| IBIS file stm32u535_545_lqfp100.ibs
[IBIS ver] 4.2
[File name] stm32u535_545_lqfp100.ibs
[File Rev] rev1.0
[Date]  11-09-2023
[Source] Data Created at STMicroelectronics
[Notes]  File originated from ELDO simulations.
[Disclaimer]  This information is for modeling purpose only and is
   not guaranteed. The information is subject to change without
   notice.
[Copyright] Copyright 2023 STMicroelectronics Inc.
|   Component stm32u535_545_lqfp100
[Component] stm32u535_545_lqfp100
[Manufacturer] STMicroelectronics
[Package]
| variable   typ   min   max
R_pkg  0  NA  NA
L_pkg  0  NA  NA
C_pkg  0  NA  NA
[Pin]   signal_name   model_name
1  PE2  io8_100m_hslv_ft
2  PE3  io8_100m_hslv_tamp_ft
3  PE4  io8_100m_hslv_tamp_ft
4  PE5  io8_100m_hslv_tamp_ft
5  PE6  io8_100m_hslv_tamp_ft
6  VBAT  power
7  PC13  io8_100m_ft_v33
8  PC14-OSC32_IN  io8_100m_tamp_ft
9  PC15-OSC32_OUT  io8_100m_tamp_ft
10  VSS  gnd
11  VDD  power
12  PH0-OSC_IN  io8_100m_ft
13  PH1-OSC_OUT  io8_100m_ft
14  NRST  nc
15  PC0  io8_100m_hslv_i2c_ft
16  PC1  io8_166m_hslv_i2c_ft
17  PC2  io8_100m_hslv_ft
18  PC3  io8_100m_hslv_ft
19  VSSA  nc
20  VREFM  nc
21  VREFP  nc
22  VDDA  power
23  PA0  io8_100m_hslv_tamp_ft
24  PA1  io8_100m_hslv_tamp_ft
25  PA2  io8_100m_hslv_ft
26  PA3  io8_166m_hslv_ft
27  VSS  gnd
28  VDD  power
29  PA4  io8_100m_hslv_ft
30  PA5  io8_100m_ft
31  PA6  io8_100m_hslv_ft
32  PA7  io8_100m_hslv_i2c_ft
33  PC4  io8_100m_hslv_ft
34  PC5  io8_100m_tamp_ft
35  PB0  io8_100m_hslv_ft
36  PB1  io8_100m_hslv_ft
37  PB2  io8_100m_hslv_tamp_ft
38  PE7  io8_100m_hslv_ft
39  PE8  io8_100m_hslv_ft
40  PE9  io8_166m_hslv_ft
41  PE10  io8_166m_hslv_ft
42  PE11  io8_100m_hslv_ft
43  PE12  io8_100m_hslv_ft
44  PE13  io8_100m_hslv_ft
45  PE14  io8_100m_hslv_ft
46  PE15  io8_100m_hslv_ft
47  PB10  io8_166m_hslv_i2c_ft
48  VCAP  nc
49  VSS  gnd
50  VDD  power
51  PB12  io8_166m_hslv_ft
52  PB13  io8_100m_i2c_ft
53  PB14  io8_100m_i2c_ft
54  PB15  io8_100m_ft
55  PD8  io8_100m_hslv_ft
56  PD9  io8_100m_hslv_ft
57  PD10  io8_100m_hslv_ft
58  PD11  io8_100m_hslv_ft
59  PD12  io8_100m_hslv_i2c_ft
60  PD13  io8_100m_hslv_i2c_ft
61  PD14  io8_100m_hslv_ft
62  PD15  io8_100m_hslv_ft
63  PC6  io8_100m_hslv_ft
64  PC7  io8_100m_hslv_ft
65  PC8  io8_100m_hslv_ft
66  PC9  io8_100m_hslv_ft
67  PA8  io8_166m_hslv_ft
68  PA9  io8_100m_ft
69  PA10  io8_100m_ft
70  PA11  io8_usb_ft
71  PA12  io8_usb_ft
72  PA13  io8_100m_ft
73  VDDUSB  power
74  VSS  gnd
75  VDD  power
76  PA14  io8_100m_ft
77  PA15  io8_100m_ft
78  PC10  io8_100m_hslv_ft
79  PC11  io8_100m_hslv_ft
80  PC12  io8_166m_hslv_ft
81  PD0  io8_100m_hslv_ft
82  PD1  io8_100m_hslv_ft
83  PD2  io8_100m_hslv_ft
84  PD3  io8_166m_hslv_ft
85  PD4  io8_100m_hslv_ft
86  PD5  io8_100m_hslv_ft
87  PD6  io8_166m_hslv_ft
88  PD7  io8_100m_hslv_ft
89  PB3  io8_100m_i2c_ft
90  PB4  io8_100m_i2c_ft
91  PB5  io8_166m_hslv_ft
92  PB6  io8_100m_i2c_ft
93  PB7  io8_166m_hslv_i2c_ft
94  PH3-BOOT0  io8_100m_ft
95  PB8  io8_100m_hslv_i2c_ft
96  PB9  io8_100m_hslv_i2c_ft
97  PE0  io8_100m_hslv_ft
98  PE1  io8_100m_hslv_ft
99  VSS  gnd
100  VDD power
[Package Model]   455-lqfp-14x14-100-ldo-230504
[Pin Mapping]   pulldown_ref   pullup_ref   | Comment
1  gndio  vddiom
2  gndio  vddiom
3  gndio  vddiom
4  gndio  vddiom
5  gndio  vddiom
6  nc  vsw
7  gndio  vddiom  | Depending on IO usage
| 7  gndio  vsw  | Depending on IO usage
8  gndio  vddiom  | Depending on IO usage
| 8  gndio  vsw  | Depending on IO usage
9  gndio  vddiom  | Depending on IO usage
| 9  gndio  vsw  | Depending on IO usage
10  gndio  nc
11  nc  vddiom
12  gndio  vddiom
13  gndio  vddiom
14  nc   nc
15  gndio  vddiom
16  gndio  vddiom
17  gndio  vddiom
18  gndio  vddiom
19  nc  nc
20  nc  nc
21  nc  nc
22  nc  vddiom
23  gndio  vddiom
24  gndio  vddiom
25  gndio  vddiom
26  gndio  vddiom
27  gndio  nc
28  nc  vddiom
29  gndio  vddiom
30  gndio  vddiom
31  gndio  vddiom
32  gndio  vddiom
33  gndio  vddiom
34  gndio  vddiom
35  gndio  vddiom
36  gndio  vddiom
37  gndio  vddiom
38  gndio  vddiom
39  gndio  vddiom
40  gndio  vddiom
41  gndio  vddiom
42  gndio  vddiom
43  gndio  vddiom
44  gndio  vddiom
45  gndio  vddiom
46  gndio  vddiom
47  gndio  vddiom
48  nc  nc
49  gndio  nc
50  nc  vddiom
51  gndio  vddiom
52  gndio  vddiom
53  gndio  vddiom
54  gndio  vddiom
55  gndio  vddiom
56  gndio  vddiom
57  gndio  vddiom
58  gndio  vddiom
59  gndio  vddiom
60  gndio  vddiom
61  gndio  vddiom
62  gndio  vddiom
63  gndio  vddiom
64  gndio  vddiom
65  gndio  vddiom
66  gndio  vddiom
67  gndio  vddiom
68  gndio  vddiom  | Depending on IO usage
| 68  gndio  vddusb  | Depending on IO usage
69  gndio  vddiom  | Depending on IO usage
| 69  gndio  vddusb  | Depending on IO usage
70  gndio  vddiom  | Depending on IO usage
| 70  gndio  vddusb  | Depending on IO usage
71  gndio  vddiom  | Depending on IO usage
| 71  gndio  vddusb  | Depending on IO usage
72  gndio  vddiom  | Depending on IO usage
| 72  gndio  vddusb  | Depending on IO usage
73  nc  vddusb
74  gndio  nc
75  nc  vddiom
76  gndio  vddiom
77  gndio  vddiom
78  gndio  vddiom
79  gndio  vddiom
80  gndio  vddiom
81  gndio  vddiom
82  gndio  vddiom
83  gndio  vddiom
84  gndio  vddiom
85  gndio  vddiom
86  gndio  vddiom
87  gndio  vddiom
88  gndio  vddiom
89  gndio  vddiom
90  gndio  vddiom
91  gndio  vddiom
92  gndio  vddiom
93  gndio  vddiom
94  gndio  vddiom
95  gndio  vddiom
96  gndio  vddiom
97  gndio  vddiom
98  gndio  vddiom
99  gndio  nc
100  nc  vddiom
[Model Selector] io8_100m_ft
io8_100m_ft_hs_1v2  "IO8_FT 100MHz high speed @ 1.2V"
io8_100m_ft_fs_1v2  "IO8_FT 100MHz fast speed @ 1.2V"
io8_100m_ft_fs_pd_1v2  "IO8_FT 100MHz fast speed @ 1.2V pulldown"
io8_100m_ft_ms_1v2  "IO8_FT 100MHz med speed @ 1.2V"
io8_100m_ft_ms_pd_1v2  "IO8_FT 100MHz med speed @ 1.2V pulldown"
io8_100m_ft_ls_1v2  "IO8_FT 100MHz low speed @ 1.2V"
io8_100m_ft_ls_pd_1v2  "IO8_FT 100MHz low speed @ 1.2V pulldown"
io8_100m_ft_hs_1v8  "IO8_FT 100MHz high speed @ 1.8V"
io8_100m_ft_hs_pd_1v8  "IO8_FT 100MHz high speed @ 1.8V pulldown"
io8_100m_ft_fs_1v8  "IO8_FT 100MHz fast speed @ 1.8V"
io8_100m_ft_fs_pd_1v8  "IO8_FT 100MHz fast speed @ 1.8V pulldown"
io8_100m_ft_ms_1v8  "IO8_FT 100MHz med speed @ 1.8V"
io8_100m_ft_ms_pd_1v8  "IO8_FT 100MHz med speed @ 1.8V pulldown"
io8_100m_ft_ls_1v8  "IO8_FT 100MHz low speed @ 1.8V"
io8_100m_ft_ls_pd_1v8  "IO8_FT 100MHz low speed @ 1.8V pulldown"
io8_100m_ft_hs_3v3  "IO8_FT 100MHz high speed @ 3.3V"
io8_100m_ft_hs_pd_3v3  "IO8_FT 100MHz high speed @ 3.3V pulldown"
io8_100m_ft_fs_3v3  "IO8_FT 100MHz fast speed @ 3.3V"
io8_100m_ft_fs_pd_3v3  "IO8_FT 100MHz fast speed @ 3.3V pulldown"
io8_100m_ft_ms_3v3  "IO8_FT 100MHz med speed @ 3.3V"
io8_100m_ft_ms_pd_3v3  "IO8_FT 100MHz med speed @ 3.3V pulldown"
io8_100m_ft_ls_3v3  "IO8_FT 100MHz low speed @ 3.3V"
io8_100m_ft_ls_pd_3v3  "IO8_FT 100MHz low speed @ 3.3V pulldown"
[Model Selector] io8_100m_hslv_ft
io8_100m_ft_hs_1v2  "IO8_FT 100MHz high speed @ 1.2V"
io8_100m_ft_hs_pu_1v2  "IO8_FT 100MHz high speed @ 1.2V pullup"
io8_100m_ft_hs_pd_1v2  "IO8_FT 100MHz high speed @ 1.2V pulldown"
io8_100m_ft_fs_1v2  "IO8_FT 100MHz fast speed @ 1.2V"
io8_100m_ft_fs_pu_1v2  "IO8_FT 100MHz fast speed @ 1.2V pullup"
io8_100m_ft_fs_pd_1v2  "IO8_FT 100MHz fast speed @ 1.2V pulldown"
io8_100m_ft_ms_1v2  "IO8_FT 100MHz med speed @ 1.2V"
io8_100m_ft_ms_pu_1v2  "IO8_FT 100MHz med speed @ 1.2V pullup"
io8_100m_ft_ms_pd_1v2  "IO8_FT 100MHz med speed @ 1.2V pulldown"
io8_100m_ft_ls_1v2  "IO8_FT 100MHz low speed @ 1.2V"
io8_100m_ft_ls_pu_1v2  "IO8_FT 100MHz low speed @ 1.2V pullup"
io8_100m_ft_ls_pd_1v2  "IO8_FT 100MHz low speed @ 1.2V pulldown"
io8_100m_ft_hs_1v8  "IO8_FT 100MHz high speed @ 1.8V"
io8_100m_ft_hs_pu_1v8  "IO8_FT 100MHz high speed @ 1.8V pullup"
io8_100m_ft_hs_pd_1v8  "IO8_FT 100MHz high speed @ 1.8V pulldown"
io8_100m_ft_fs_1v8  "IO8_FT 100MHz fast speed @ 1.8V"
io8_100m_ft_fs_pu_1v8  "IO8_FT 100MHz fast speed @ 1.8V pullup"
io8_100m_ft_fs_pd_1v8  "IO8_FT 100MHz fast speed @ 1.8V pulldown"
io8_100m_ft_ms_1v8  "IO8_FT 100MHz med speed @ 1.8V"
io8_100m_ft_ms_pu_1v8  "IO8_FT 100MHz med speed @ 1.8V pullup"
io8_100m_ft_ms_pd_1v8  "IO8_FT 100MHz med speed @ 1.8V pulldown"
io8_100m_ft_ls_1v8  "IO8_FT 100MHz low speed @ 1.8V"
io8_100m_ft_ls_pu_1v8  "IO8_FT 100MHz low speed @ 1.8V pullup"
io8_100m_ft_ls_pd_1v8  "IO8_FT 100MHz low speed @ 1.8V pulldown"
io8_100m_ft_hs_3v3  "IO8_FT 100MHz high speed @ 3.3V"
io8_100m_ft_hs_pu_3v3  "IO8_FT 100MHz high speed @ 3.3V pullup"
io8_100m_ft_hs_pd_3v3  "IO8_FT 100MHz high speed @ 3.3V pulldown"
io8_100m_ft_fs_3v3  "IO8_FT 100MHz fast speed @ 3.3V"
io8_100m_ft_fs_pu_3v3  "IO8_FT 100MHz fast speed @ 3.3V pullup"
io8_100m_ft_fs_pd_3v3  "IO8_FT 100MHz fast speed @ 3.3V pulldown"
io8_100m_ft_ms_3v3  "IO8_FT 100MHz med speed @ 3.3V"
io8_100m_ft_ms_pu_3v3  "IO8_FT 100MHz med speed @ 3.3V pullup"
io8_100m_ft_ms_pd_3v3  "IO8_FT 100MHz med speed @ 3.3V pulldown"
io8_100m_ft_ls_3v3  "IO8_FT 100MHz low speed @ 3.3V"
io8_100m_ft_ls_pu_3v3  "IO8_FT 100MHz low speed @ 3.3V pullup"
io8_100m_ft_ls_pd_3v3  "IO8_FT 100MHz low speed @ 3.3V pulldown"
io8_100m_hslv_ft_hs_1v2  "IO8_FT 100MHz HSLV high speed @ 1.2V"
io8_100m_hslv_ft_hs_pu_1v2  "IO8_FT 100MHz HSLV high speed @ 1.2V pullup"
io8_100m_hslv_ft_hs_pd_1v2  "IO8_FT 100MHz HSLV high speed @ 1.2V pulldown"
io8_100m_hslv_ft_fs_1v2  "IO8_FT 100MHz HSLV fast speed @ 1.2V"
io8_100m_hslv_ft_fs_pu_1v2  "IO8_FT 100MHz HSLV fast speed @ 1.2V pullup"
io8_100m_hslv_ft_fs_pd_1v2  "IO8_FT 100MHz HSLV fast speed @ 1.2V pulldown"
io8_100m_hslv_ft_ms_1v2  "IO8_FT 100MHz HSLV med speed @ 1.2V"
io8_100m_hslv_ft_ms_pu_1v2  "IO8_FT 100MHz HSLV med speed @ 1.2V pullup"
io8_100m_hslv_ft_ms_pd_1v2  "IO8_FT 100MHz HSLV med speed @ 1.2V pulldown"
io8_100m_hslv_ft_ls_1v2  "IO8_FT 100MHz HSLV low speed @ 1.2V"
io8_100m_hslv_ft_ls_pu_1v2  "IO8_FT 100MHz HSLV low speed @ 1.2V pullup"
io8_100m_hslv_ft_ls_pd_1v2  "IO8_FT 100MHz HSLV low speed @ 1.2V pulldown"
io8_100m_hslv_ft_hs_1v8  "IO8_FT 100MHz HSLV high speed @ 1.8V"
io8_100m_hslv_ft_hs_pu_1v8  "IO8_FT 100MHz HSLV high speed @ 1.8V pullup"
io8_100m_hslv_ft_hs_pd_1v8  "IO8_FT 100MHz HSLV high speed @ 1.8V pulldown"
io8_100m_hslv_ft_fs_1v8  "IO8_FT 100MHz HSLV fast speed @ 1.8V"
io8_100m_hslv_ft_fs_pu_1v8  "IO8_FT 100MHz HSLV fast speed @ 1.8V pullup"
io8_100m_hslv_ft_fs_pd_1v8  "IO8_FT 100MHz HSLV fast speed @ 1.8V pulldown"
io8_100m_hslv_ft_ms_1v8  "IO8_FT 100MHz HSLV med speed @ 1.8V"
io8_100m_hslv_ft_ms_pu_1v8  "IO8_FT 100MHz HSLV med speed @ 1.8V pullup"
io8_100m_hslv_ft_ms_pd_1v8  "IO8_FT 100MHz HSLV med speed @ 1.8V pulldown"
io8_100m_hslv_ft_ls_1v8  "IO8_FT 100MHz HSLV low speed @ 1.8V"
io8_100m_hslv_ft_ls_pu_1v8  "IO8_FT 100MHz HSLV low speed @ 1.8V pullup"
io8_100m_hslv_ft_ls_pd_1v8  "IO8_FT 100MHz HSLV low speed @ 1.8V pulldown"
io8_100m_hslv_ft_hs_2v5  "IO8_FT 100MHz HSLV high speed @ 2.5V"
io8_100m_hslv_ft_hs_pu_2v5  "IO8_FT 100MHz HSLV high speed @ 2.5V pullup"
io8_100m_hslv_ft_hs_pd_2v5  "IO8_FT 100MHz HSLV high speed @ 2.5V pulldown"
io8_100m_hslv_ft_fs_2v5  "IO8_FT 100MHz HSLV fast speed @ 2.5V"
io8_100m_hslv_ft_fs_pu_2v5  "IO8_FT 100MHz HSLV fast speed @ 2.5V pullup"
io8_100m_hslv_ft_fs_pd_2v5  "IO8_FT 100MHz HSLV fast speed @ 2.5V pulldown"
io8_100m_hslv_ft_ms_2v5  "IO8_FT 100MHz HSLV med speed @ 2.5V"
io8_100m_hslv_ft_ms_pu_2v5  "IO8_FT 100MHz HSLV med speed @ 2.5V pullup"
io8_100m_hslv_ft_ms_pd_2v5  "IO8_FT 100MHz HSLV med speed @ 2.5V pulldown"
io8_100m_hslv_ft_ls_2v5  "IO8_FT 100MHz HSLV low speed @ 2.5V"
io8_100m_hslv_ft_ls_pu_2v5  "IO8_FT 100MHz HSLV low speed @ 2.5V pullup"
io8_100m_hslv_ft_ls_pd_2v5  "IO8_FT 100MHz HSLV low speed @ 2.5V pulldown"
[Model Selector] io8_100m_hslv_i2c_ft
io8_100m_ft_hs_1v2  "IO8_FT 100MHz high speed @ 1.2V"
io8_100m_ft_hs_pu_1v2  "IO8_FT 100MHz high speed @ 1.2V pullup"
io8_100m_ft_hs_pd_1v2  "IO8_FT 100MHz high speed @ 1.2V pulldown"
io8_100m_ft_fs_1v2  "IO8_FT 100MHz fast speed @ 1.2V"
io8_100m_ft_fs_pu_1v2  "IO8_FT 100MHz fast speed @ 1.2V pullup"
io8_100m_ft_fs_pd_1v2  "IO8_FT 100MHz fast speed @ 1.2V pulldown"
io8_100m_ft_ms_1v2  "IO8_FT 100MHz med speed @ 1.2V"
io8_100m_ft_ms_pu_1v2  "IO8_FT 100MHz med speed @ 1.2V pullup"
io8_100m_ft_ms_pd_1v2  "IO8_FT 100MHz med speed @ 1.2V pulldown"
io8_100m_ft_ls_1v2  "IO8_FT 100MHz low speed @ 1.2V"
io8_100m_ft_ls_pu_1v2  "IO8_FT 100MHz low speed @ 1.2V pullup"
io8_100m_ft_ls_pd_1v2  "IO8_FT 100MHz low speed @ 1.2V pulldown"
io8_100m_ft_hs_1v8  "IO8_FT 100MHz high speed @ 1.8V"
io8_100m_ft_hs_pu_1v8  "IO8_FT 100MHz high speed @ 1.8V pullup"
io8_100m_ft_hs_pd_1v8  "IO8_FT 100MHz high speed @ 1.8V pulldown"
io8_100m_ft_fs_1v8  "IO8_FT 100MHz fast speed @ 1.8V"
io8_100m_ft_fs_pu_1v8  "IO8_FT 100MHz fast speed @ 1.8V pullup"
io8_100m_ft_fs_pd_1v8  "IO8_FT 100MHz fast speed @ 1.8V pulldown"
io8_100m_ft_ms_1v8  "IO8_FT 100MHz med speed @ 1.8V"
io8_100m_ft_ms_pu_1v8  "IO8_FT 100MHz med speed @ 1.8V pullup"
io8_100m_ft_ms_pd_1v8  "IO8_FT 100MHz med speed @ 1.8V pulldown"
io8_100m_ft_ls_1v8  "IO8_FT 100MHz low speed @ 1.8V"
io8_100m_ft_ls_pu_1v8  "IO8_FT 100MHz low speed @ 1.8V pullup"
io8_100m_ft_ls_pd_1v8  "IO8_FT 100MHz low speed @ 1.8V pulldown"
io8_100m_ft_hs_3v3  "IO8_FT 100MHz high speed @ 3.3V"
io8_100m_ft_hs_pu_3v3  "IO8_FT 100MHz high speed @ 3.3V pullup"
io8_100m_ft_hs_pd_3v3  "IO8_FT 100MHz high speed @ 3.3V pulldown"
io8_100m_ft_fs_3v3  "IO8_FT 100MHz fast speed @ 3.3V"
io8_100m_ft_fs_pu_3v3  "IO8_FT 100MHz fast speed @ 3.3V pullup"
io8_100m_ft_fs_pd_3v3  "IO8_FT 100MHz fast speed @ 3.3V pulldown"
io8_100m_ft_ms_3v3  "IO8_FT 100MHz med speed @ 3.3V"
io8_100m_ft_ms_pu_3v3  "IO8_FT 100MHz med speed @ 3.3V pullup"
io8_100m_ft_ms_pd_3v3  "IO8_FT 100MHz med speed @ 3.3V pulldown"
io8_100m_ft_ls_3v3  "IO8_FT 100MHz low speed @ 3.3V"
io8_100m_ft_ls_pu_3v3  "IO8_FT 100MHz low speed @ 3.3V pullup"
io8_100m_ft_ls_pd_3v3  "IO8_FT 100MHz low speed @ 3.3V pulldown"
io8_100m_hslv_ft_hs_1v2  "IO8_FT 100MHz HSLV high speed @ 1.2V"
io8_100m_hslv_ft_hs_pu_1v2  "IO8_FT 100MHz HSLV high speed @ 1.2V pullup"
io8_100m_hslv_ft_hs_pd_1v2  "IO8_FT 100MHz HSLV high speed @ 1.2V pulldown"
io8_100m_hslv_ft_fs_1v2  "IO8_FT 100MHz HSLV fast speed @ 1.2V"
io8_100m_hslv_ft_fs_pu_1v2  "IO8_FT 100MHz HSLV fast speed @ 1.2V pullup"
io8_100m_hslv_ft_fs_pd_1v2  "IO8_FT 100MHz HSLV fast speed @ 1.2V pulldown"
io8_100m_hslv_ft_ms_1v2  "IO8_FT 100MHz HSLV med speed @ 1.2V"
io8_100m_hslv_ft_ms_pu_1v2  "IO8_FT 100MHz HSLV med speed @ 1.2V pullup"
io8_100m_hslv_ft_ms_pd_1v2  "IO8_FT 100MHz HSLV med speed @ 1.2V pulldown"
io8_100m_hslv_ft_ls_1v2  "IO8_FT 100MHz HSLV low speed @ 1.2V"
io8_100m_hslv_ft_ls_pu_1v2  "IO8_FT 100MHz HSLV low speed @ 1.2V pullup"
io8_100m_hslv_ft_ls_pd_1v2  "IO8_FT 100MHz HSLV low speed @ 1.2V pulldown"
io8_100m_hslv_ft_hs_1v8  "IO8_FT 100MHz HSLV high speed @ 1.8V"
io8_100m_hslv_ft_hs_pu_1v8  "IO8_FT 100MHz HSLV high speed @ 1.8V pullup"
io8_100m_hslv_ft_hs_pd_1v8  "IO8_FT 100MHz HSLV high speed @ 1.8V pulldown"
io8_100m_hslv_ft_fs_1v8  "IO8_FT 100MHz HSLV fast speed @ 1.8V"
io8_100m_hslv_ft_fs_pu_1v8  "IO8_FT 100MHz HSLV fast speed @ 1.8V pullup"
io8_100m_hslv_ft_fs_pd_1v8  "IO8_FT 100MHz HSLV fast speed @ 1.8V pulldown"
io8_100m_hslv_ft_ms_1v8  "IO8_FT 100MHz HSLV med speed @ 1.8V"
io8_100m_hslv_ft_ms_pu_1v8  "IO8_FT 100MHz HSLV med speed @ 1.8V pullup"
io8_100m_hslv_ft_ms_pd_1v8  "IO8_FT 100MHz HSLV med speed @ 1.8V pulldown"
io8_100m_hslv_ft_ls_1v8  "IO8_FT 100MHz HSLV low speed @ 1.8V"
io8_100m_hslv_ft_ls_pu_1v8  "IO8_FT 100MHz HSLV low speed @ 1.8V pullup"
io8_100m_hslv_ft_ls_pd_1v8  "IO8_FT 100MHz HSLV low speed @ 1.8V pulldown"
io8_100m_hslv_ft_hs_2v5  "IO8_FT 100MHz HSLV high speed @ 2.5V"
io8_100m_hslv_ft_hs_pu_2v5  "IO8_FT 100MHz HSLV high speed @ 2.5V pullup"
io8_100m_hslv_ft_hs_pd_2v5  "IO8_FT 100MHz HSLV high speed @ 2.5V pulldown"
io8_100m_hslv_ft_fs_2v5  "IO8_FT 100MHz HSLV fast speed @ 2.5V"
io8_100m_hslv_ft_fs_pu_2v5  "IO8_FT 100MHz HSLV fast speed @ 2.5V pullup"
io8_100m_hslv_ft_fs_pd_2v5  "IO8_FT 100MHz HSLV fast speed @ 2.5V pulldown"
io8_100m_hslv_ft_ms_2v5  "IO8_FT 100MHz HSLV med speed @ 2.5V"
io8_100m_hslv_ft_ms_pu_2v5  "IO8_FT 100MHz HSLV med speed @ 2.5V pullup"
io8_100m_hslv_ft_ms_pd_2v5  "IO8_FT 100MHz HSLV med speed @ 2.5V pulldown"
io8_100m_hslv_ft_ls_2v5  "IO8_FT 100MHz HSLV low speed @ 2.5V"
io8_100m_hslv_ft_ls_pu_2v5  "IO8_FT 100MHz HSLV low speed @ 2.5V pullup"
io8_100m_hslv_ft_ls_pd_2v5  "IO8_FT 100MHz HSLV low speed @ 2.5V pulldown"
[Model Selector] io8_100m_hslv_tamp_ft
io8_100m_ft_hs_1v2  "IO8_FT 100MHz high speed @ 1.2V"
io8_100m_ft_hs_pu_1v2  "IO8_FT 100MHz high speed @ 1.2V pullup"
io8_100m_ft_hs_pd_1v2  "IO8_FT 100MHz high speed @ 1.2V pulldown"
io8_100m_ft_fs_1v2  "IO8_FT 100MHz fast speed @ 1.2V"
io8_100m_ft_fs_pu_1v2  "IO8_FT 100MHz fast speed @ 1.2V pullup"
io8_100m_ft_fs_pd_1v2  "IO8_FT 100MHz fast speed @ 1.2V pulldown"
io8_100m_ft_ms_1v2  "IO8_FT 100MHz med speed @ 1.2V"
io8_100m_ft_ms_pu_1v2  "IO8_FT 100MHz med speed @ 1.2V pullup"
io8_100m_ft_ms_pd_1v2  "IO8_FT 100MHz med speed @ 1.2V pulldown"
io8_100m_ft_ls_1v2  "IO8_FT 100MHz low speed @ 1.2V"
io8_100m_ft_ls_pu_1v2  "IO8_FT 100MHz low speed @ 1.2V pullup"
io8_100m_ft_ls_pd_1v2  "IO8_FT 100MHz low speed @ 1.2V pulldown"
io8_100m_ft_hs_1v8  "IO8_FT 100MHz high speed @ 1.8V"
io8_100m_ft_hs_pu_1v8  "IO8_FT 100MHz high speed @ 1.8V pullup"
io8_100m_ft_hs_pd_1v8  "IO8_FT 100MHz high speed @ 1.8V pulldown"
io8_100m_ft_fs_1v8  "IO8_FT 100MHz fast speed @ 1.8V"
io8_100m_ft_fs_pu_1v8  "IO8_FT 100MHz fast speed @ 1.8V pullup"
io8_100m_ft_fs_pd_1v8  "IO8_FT 100MHz fast speed @ 1.8V pulldown"
io8_100m_ft_ms_1v8  "IO8_FT 100MHz med speed @ 1.8V"
io8_100m_ft_ms_pu_1v8  "IO8_FT 100MHz med speed @ 1.8V pullup"
io8_100m_ft_ms_pd_1v8  "IO8_FT 100MHz med speed @ 1.8V pulldown"
io8_100m_ft_ls_1v8  "IO8_FT 100MHz low speed @ 1.8V"
io8_100m_ft_ls_pu_1v8  "IO8_FT 100MHz low speed @ 1.8V pullup"
io8_100m_ft_ls_pd_1v8  "IO8_FT 100MHz low speed @ 1.8V pulldown"
io8_100m_ft_hs_3v3  "IO8_FT 100MHz high speed @ 3.3V"
io8_100m_ft_hs_pu_3v3  "IO8_FT 100MHz high speed @ 3.3V pullup"
io8_100m_ft_hs_pd_3v3  "IO8_FT 100MHz high speed @ 3.3V pulldown"
io8_100m_ft_fs_3v3  "IO8_FT 100MHz fast speed @ 3.3V"
io8_100m_ft_fs_pu_3v3  "IO8_FT 100MHz fast speed @ 3.3V pullup"
io8_100m_ft_fs_pd_3v3  "IO8_FT 100MHz fast speed @ 3.3V pulldown"
io8_100m_ft_ms_3v3  "IO8_FT 100MHz med speed @ 3.3V"
io8_100m_ft_ms_pu_3v3  "IO8_FT 100MHz med speed @ 3.3V pullup"
io8_100m_ft_ms_pd_3v3  "IO8_FT 100MHz med speed @ 3.3V pulldown"
io8_100m_ft_ls_3v3  "IO8_FT 100MHz low speed @ 3.3V"
io8_100m_ft_ls_pu_3v3  "IO8_FT 100MHz low speed @ 3.3V pullup"
io8_100m_ft_ls_pd_3v3  "IO8_FT 100MHz low speed @ 3.3V pulldown"
io8_100m_hslv_ft_hs_1v2  "IO8_FT 100MHz HSLV high speed @ 1.2V"
io8_100m_hslv_ft_hs_pu_1v2  "IO8_FT 100MHz HSLV high speed @ 1.2V pullup"
io8_100m_hslv_ft_hs_pd_1v2  "IO8_FT 100MHz HSLV high speed @ 1.2V pulldown"
io8_100m_hslv_ft_fs_1v2  "IO8_FT 100MHz HSLV fast speed @ 1.2V"
io8_100m_hslv_ft_fs_pu_1v2  "IO8_FT 100MHz HSLV fast speed @ 1.2V pullup"
io8_100m_hslv_ft_fs_pd_1v2  "IO8_FT 100MHz HSLV fast speed @ 1.2V pulldown"
io8_100m_hslv_ft_ms_1v2  "IO8_FT 100MHz HSLV med speed @ 1.2V"
io8_100m_hslv_ft_ms_pu_1v2  "IO8_FT 100MHz HSLV med speed @ 1.2V pullup"
io8_100m_hslv_ft_ms_pd_1v2  "IO8_FT 100MHz HSLV med speed @ 1.2V pulldown"
io8_100m_hslv_ft_ls_1v2  "IO8_FT 100MHz HSLV low speed @ 1.2V"
io8_100m_hslv_ft_ls_pu_1v2  "IO8_FT 100MHz HSLV low speed @ 1.2V pullup"
io8_100m_hslv_ft_ls_pd_1v2  "IO8_FT 100MHz HSLV low speed @ 1.2V pulldown"
io8_100m_hslv_ft_hs_1v8  "IO8_FT 100MHz HSLV high speed @ 1.8V"
io8_100m_hslv_ft_hs_pu_1v8  "IO8_FT 100MHz HSLV high speed @ 1.8V pullup"
io8_100m_hslv_ft_hs_pd_1v8  "IO8_FT 100MHz HSLV high speed @ 1.8V pulldown"
io8_100m_hslv_ft_fs_1v8  "IO8_FT 100MHz HSLV fast speed @ 1.8V"
io8_100m_hslv_ft_fs_pu_1v8  "IO8_FT 100MHz HSLV fast speed @ 1.8V pullup"
io8_100m_hslv_ft_fs_pd_1v8  "IO8_FT 100MHz HSLV fast speed @ 1.8V pulldown"
io8_100m_hslv_ft_ms_1v8  "IO8_FT 100MHz HSLV med speed @ 1.8V"
io8_100m_hslv_ft_ms_pu_1v8  "IO8_FT 100MHz HSLV med speed @ 1.8V pullup"
io8_100m_hslv_ft_ms_pd_1v8  "IO8_FT 100MHz HSLV med speed @ 1.8V pulldown"
io8_100m_hslv_ft_ls_1v8  "IO8_FT 100MHz HSLV low speed @ 1.8V"
io8_100m_hslv_ft_ls_pu_1v8  "IO8_FT 100MHz HSLV low speed @ 1.8V pullup"
io8_100m_hslv_ft_ls_pd_1v8  "IO8_FT 100MHz HSLV low speed @ 1.8V pulldown"
io8_100m_hslv_ft_hs_2v5  "IO8_FT 100MHz HSLV high speed @ 2.5V"
io8_100m_hslv_ft_hs_pu_2v5  "IO8_FT 100MHz HSLV high speed @ 2.5V pullup"
io8_100m_hslv_ft_hs_pd_2v5  "IO8_FT 100MHz HSLV high speed @ 2.5V pulldown"
io8_100m_hslv_ft_fs_2v5  "IO8_FT 100MHz HSLV fast speed @ 2.5V"
io8_100m_hslv_ft_fs_pu_2v5  "IO8_FT 100MHz HSLV fast speed @ 2.5V pullup"
io8_100m_hslv_ft_fs_pd_2v5  "IO8_FT 100MHz HSLV fast speed @ 2.5V pulldown"
io8_100m_hslv_ft_ms_2v5  "IO8_FT 100MHz HSLV med speed @ 2.5V"
io8_100m_hslv_ft_ms_pu_2v5  "IO8_FT 100MHz HSLV med speed @ 2.5V pullup"
io8_100m_hslv_ft_ms_pd_2v5  "IO8_FT 100MHz HSLV med speed @ 2.5V pulldown"
io8_100m_hslv_ft_ls_2v5  "IO8_FT 100MHz HSLV low speed @ 2.5V"
io8_100m_hslv_ft_ls_pu_2v5  "IO8_FT 100MHz HSLV low speed @ 2.5V pullup"
io8_100m_hslv_ft_ls_pd_2v5  "IO8_FT 100MHz HSLV low speed @ 2.5V pulldown"
io8_ft_v33_hs_1v2  "IO8_FT_V33 high speed @ 1.2V"
io8_ft_v33_hs_pu_1v2  "IO8_FT_V33 high speed @ 1.2V pullup"
io8_ft_v33_hs_pd_1v2  "IO8_FT_V33 high speed @ 1.2V pulldown"
io8_ft_v33_fs_1v2  "IO8_FT_V33 fast speed @ 1.2V"
io8_ft_v33_fs_pu_1v2  "IO8_FT_V33 fast speed @ 1.2V pullup"
io8_ft_v33_fs_pd_1v2  "IO8_FT_V33 fast speed @ 1.2V pulldown"
io8_ft_v33_ms_1v2  "IO8_FT_V33 med speed @ 1.2V"
io8_ft_v33_ms_pu_1v2  "IO8_FT_V33 med speed @ 1.2V pullup"
io8_ft_v33_ms_pd_1v2  "IO8_FT_V33 med speed @ 1.2V pulldown"
io8_ft_v33_ls_1v2  "IO8_FT_V33 low speed @ 1.2V"
io8_ft_v33_ls_pu_1v2  "IO8_FT_V33 low speed @ 1.2V pullup"
io8_ft_v33_ls_pd_1v2  "IO8_FT_V33 low speed @ 1.2V pulldown"
io8_ft_v33_hs_1v8  "IO8_FT_V33 high speed @ 1.8V"
io8_ft_v33_hs_pu_1v8  "IO8_FT_V33 high speed @ 1.8V pullup"
io8_ft_v33_hs_pd_1v8  "IO8_FT_V33 high speed @ 1.8V pulldown"
io8_ft_v33_fs_1v8  "IO8_FT_V33 fast speed @ 1.8V"
io8_ft_v33_fs_pu_1v8  "IO8_FT_V33 fast speed @ 1.8V pullup"
io8_ft_v33_fs_pd_1v8  "IO8_FT_V33 fast speed @ 1.8V pulldown"
io8_ft_v33_ms_1v8  "IO8_FT_V33 med speed @ 1.8V"
io8_ft_v33_ms_pu_1v8  "IO8_FT_V33 med speed @ 1.8V pullup"
io8_ft_v33_ms_pd_1v8  "IO8_FT_V33 med speed @ 1.8V pulldown"
io8_ft_v33_ls_1v8  "IO8_FT_V33 low speed @ 1.8V"
io8_ft_v33_ls_pu_1v8  "IO8_FT_V33 low speed @ 1.8V pullup"
io8_ft_v33_ls_pd_1v8  "IO8_FT_V33 low speed @ 1.8V pulldown"
io8_ft_v33_hs_3v3  "IO8_FT_V33 high speed @ 3.3V"
io8_ft_v33_hs_pu_3v3  "IO8_FT_V33 high speed @ 3.3V pullup"
io8_ft_v33_hs_pd_3v3  "IO8_FT_V33 high speed @ 3.3V pulldown"
io8_ft_v33_fs_3v3  "IO8_FT_V33 fast speed @ 3.3V"
io8_ft_v33_fs_pu_3v3  "IO8_FT_V33 fast speed @ 3.3V pullup"
io8_ft_v33_fs_pd_3v3  "IO8_FT_V33 fast speed @ 3.3V pulldown"
io8_ft_v33_ms_3v3  "IO8_FT_V33 med speed @ 3.3V"
io8_ft_v33_ms_pu_3v3  "IO8_FT_V33 med speed @ 3.3V pullup"
io8_ft_v33_ms_pd_3v3  "IO8_FT_V33 med speed @ 3.3V pulldown"
io8_ft_v33_ls_3v3  "IO8_FT_V33 low speed @ 3.3V"
io8_ft_v33_ls_pu_3v3  "IO8_FT_V33 low speed @ 3.3V pullup"
io8_ft_v33_ls_pd_3v3  "IO8_FT_V33 low speed @ 3.3V pulldown"
[Model Selector] io8_100m_i2c_ft
io8_100m_ft_hs_1v2  "IO8_FT 100MHz high speed @ 1.2V"
io8_100m_ft_hs_pu_1v2  "IO8_FT 100MHz high speed @ 1.2V pullup"
io8_100m_ft_hs_pd_1v2  "IO8_FT 100MHz high speed @ 1.2V pulldown"
io8_100m_ft_fs_1v2  "IO8_FT 100MHz fast speed @ 1.2V"
io8_100m_ft_fs_pu_1v2  "IO8_FT 100MHz fast speed @ 1.2V pullup"
io8_100m_ft_fs_pd_1v2  "IO8_FT 100MHz fast speed @ 1.2V pulldown"
io8_100m_ft_ms_1v2  "IO8_FT 100MHz med speed @ 1.2V"
io8_100m_ft_ms_pu_1v2  "IO8_FT 100MHz med speed @ 1.2V pullup"
io8_100m_ft_ms_pd_1v2  "IO8_FT 100MHz med speed @ 1.2V pulldown"
io8_100m_ft_ls_1v2  "IO8_FT 100MHz low speed @ 1.2V"
io8_100m_ft_ls_pu_1v2  "IO8_FT 100MHz low speed @ 1.2V pullup"
io8_100m_ft_ls_pd_1v2  "IO8_FT 100MHz low speed @ 1.2V pulldown"
io8_100m_ft_hs_1v8  "IO8_FT 100MHz high speed @ 1.8V"
io8_100m_ft_hs_pu_1v8  "IO8_FT 100MHz high speed @ 1.8V pullup"
io8_100m_ft_hs_pd_1v8  "IO8_FT 100MHz high speed @ 1.8V pulldown"
io8_100m_ft_fs_1v8  "IO8_FT 100MHz fast speed @ 1.8V"
io8_100m_ft_fs_pu_1v8  "IO8_FT 100MHz fast speed @ 1.8V pullup"
io8_100m_ft_fs_pd_1v8  "IO8_FT 100MHz fast speed @ 1.8V pulldown"
io8_100m_ft_ms_1v8  "IO8_FT 100MHz med speed @ 1.8V"
io8_100m_ft_ms_pu_1v8  "IO8_FT 100MHz med speed @ 1.8V pullup"
io8_100m_ft_ms_pd_1v8  "IO8_FT 100MHz med speed @ 1.8V pulldown"
io8_100m_ft_ls_1v8  "IO8_FT 100MHz low speed @ 1.8V"
io8_100m_ft_ls_pu_1v8  "IO8_FT 100MHz low speed @ 1.8V pullup"
io8_100m_ft_ls_pd_1v8  "IO8_FT 100MHz low speed @ 1.8V pulldown"
io8_100m_ft_hs_3v3  "IO8_FT 100MHz high speed @ 3.3V"
io8_100m_ft_hs_pu_3v3  "IO8_FT 100MHz high speed @ 3.3V pullup"
io8_100m_ft_hs_pd_3v3  "IO8_FT 100MHz high speed @ 3.3V pulldown"
io8_100m_ft_fs_3v3  "IO8_FT 100MHz fast speed @ 3.3V"
io8_100m_ft_fs_pu_3v3  "IO8_FT 100MHz fast speed @ 3.3V pullup"
io8_100m_ft_fs_pd_3v3  "IO8_FT 100MHz fast speed @ 3.3V pulldown"
io8_100m_ft_ms_3v3  "IO8_FT 100MHz med speed @ 3.3V"
io8_100m_ft_ms_pu_3v3  "IO8_FT 100MHz med speed @ 3.3V pullup"
io8_100m_ft_ms_pd_3v3  "IO8_FT 100MHz med speed @ 3.3V pulldown"
io8_100m_ft_ls_3v3  "IO8_FT 100MHz low speed @ 3.3V"
io8_100m_ft_ls_pu_3v3  "IO8_FT 100MHz low speed @ 3.3V pullup"
io8_100m_ft_ls_pd_3v3  "IO8_FT 100MHz low speed @ 3.3V pulldown"
io8_100m_i2c_ft_1v2  "IO8_FT 100MHz I2C @ 1.2V"
io8_100m_i2c_ft_pu_1v2  "IO8_FT 100MHz I2C @ 1.2V pullup"
io8_100m_i2c_ft_pd_1v2  "IO8_FT 100MHz I2C @ 1.2V pulldown"
io8_100m_i2c_ft_1v8  "IO8_FT 100MHz I2C @ 1.8V"
io8_100m_i2c_ft_pu_1v8  "IO8_FT 100MHz I2C @ 1.8V pullup"
io8_100m_i2c_ft_pd_1v8  "IO8_FT 100MHz I2C @ 1,8V pulldown"
io8_100m_i2c_ft_3v3  "IO8_FT 100MHz I2C @ 3.3V"
io8_100m_i2c_ft_pu_3v3  "IO8_FT 100MHz I2C HSLV @ 3.3V pullup"
io8_100m_i2c_ft_pd_3v3  "IO8_FT 100MHz I2C @ 3.3V pulldown"
[Model Selector] io8_100m_tamp_ft
io8_100m_ft_hs_1v2  "IO8_FT 100MHz high speed @ 1.2V"
io8_100m_ft_hs_pu_1v2  "IO8_FT 100MHz high speed @ 1.2V pullup"
io8_100m_ft_hs_pd_1v2  "IO8_FT 100MHz high speed @ 1.2V pulldown"
io8_100m_ft_fs_1v2  "IO8_FT 100MHz fast speed @ 1.2V"
io8_100m_ft_fs_pu_1v2  "IO8_FT 100MHz fast speed @ 1.2V pullup"
io8_100m_ft_fs_pd_1v2  "IO8_FT 100MHz fast speed @ 1.2V pulldown"
io8_100m_ft_ms_1v2  "IO8_FT 100MHz med speed @ 1.2V"
io8_100m_ft_ms_pu_1v2  "IO8_FT 100MHz med speed @ 1.2V pullup"
io8_100m_ft_ms_pd_1v2  "IO8_FT 100MHz med speed @ 1.2V pulldown"
io8_100m_ft_ls_1v2  "IO8_FT 100MHz low speed @ 1.2V"
io8_100m_ft_ls_pu_1v2  "IO8_FT 100MHz low speed @ 1.2V pullup"
io8_100m_ft_ls_pd_1v2  "IO8_FT 100MHz low speed @ 1.2V pulldown"
io8_100m_ft_hs_1v8  "IO8_FT 100MHz high speed @ 1.8V"
io8_100m_ft_hs_pu_1v8  "IO8_FT 100MHz high speed @ 1.8V pullup"
io8_100m_ft_hs_pd_1v8  "IO8_FT 100MHz high speed @ 1.8V pulldown"
io8_100m_ft_fs_1v8  "IO8_FT 100MHz fast speed @ 1.8V"
io8_100m_ft_fs_pu_1v8  "IO8_FT 100MHz fast speed @ 1.8V pullup"
io8_100m_ft_fs_pd_1v8  "IO8_FT 100MHz fast speed @ 1.8V pulldown"
io8_100m_ft_ms_1v8  "IO8_FT 100MHz med speed @ 1.8V"
io8_100m_ft_ms_pu_1v8  "IO8_FT 100MHz med speed @ 1.8V pullup"
io8_100m_ft_ms_pd_1v8  "IO8_FT 100MHz med speed @ 1.8V pulldown"
io8_100m_ft_ls_1v8  "IO8_FT 100MHz low speed @ 1.8V"
io8_100m_ft_ls_pu_1v8  "IO8_FT 100MHz low speed @ 1.8V pullup"
io8_100m_ft_ls_pd_1v8  "IO8_FT 100MHz low speed @ 1.8V pulldown"
io8_100m_ft_hs_3v3  "IO8_FT 100MHz high speed @ 3.3V"
io8_100m_ft_hs_pu_3v3  "IO8_FT 100MHz high speed @ 3.3V pullup"
io8_100m_ft_hs_pd_3v3  "IO8_FT 100MHz high speed @ 3.3V pulldown"
io8_100m_ft_fs_3v3  "IO8_FT 100MHz fast speed @ 3.3V"
io8_100m_ft_fs_pu_3v3  "IO8_FT 100MHz fast speed @ 3.3V pullup"
io8_100m_ft_fs_pd_3v3  "IO8_FT 100MHz fast speed @ 3.3V pulldown"
io8_100m_ft_ms_3v3  "IO8_FT 100MHz med speed @ 3.3V"
io8_100m_ft_ms_pu_3v3  "IO8_FT 100MHz med speed @ 3.3V pullup"
io8_100m_ft_ms_pd_3v3  "IO8_FT 100MHz med speed @ 3.3V pulldown"
io8_100m_ft_ls_3v3  "IO8_FT 100MHz low speed @ 3.3V"
io8_100m_ft_ls_pu_3v3  "IO8_FT 100MHz low speed @ 3.3V pullup"
io8_100m_ft_ls_pd_3v3  "IO8_FT 100MHz low speed @ 3.3V pulldown"
io8_ft_v33_hs_1v2  "IO8_FT_V33 high speed @ 1.2V"
io8_ft_v33_hs_pu_1v2  "IO8_FT_V33 high speed @ 1.2V pullup"
io8_ft_v33_hs_pd_1v2  "IO8_FT_V33 high speed @ 1.2V pulldown"
io8_ft_v33_fs_1v2  "IO8_FT_V33 fast speed @ 1.2V"
io8_ft_v33_fs_pu_1v2  "IO8_FT_V33 fast speed @ 1.2V pullup"
io8_ft_v33_fs_pd_1v2  "IO8_FT_V33 fast speed @ 1.2V pulldown"
io8_ft_v33_ms_1v2  "IO8_FT_V33 med speed @ 1.2V"
io8_ft_v33_ms_pu_1v2  "IO8_FT_V33 med speed @ 1.2V pullup"
io8_ft_v33_ms_pd_1v2  "IO8_FT_V33 med speed @ 1.2V pulldown"
io8_ft_v33_ls_1v2  "IO8_FT_V33 low speed @ 1.2V"
io8_ft_v33_ls_pu_1v2  "IO8_FT_V33 low speed @ 1.2V pullup"
io8_ft_v33_ls_pd_1v2  "IO8_FT_V33 low speed @ 1.2V pulldown"
io8_ft_v33_hs_1v8  "IO8_FT_V33 high speed @ 1.8V"
io8_ft_v33_hs_pu_1v8  "IO8_FT_V33 high speed @ 1.8V pullup"
io8_ft_v33_hs_pd_1v8  "IO8_FT_V33 high speed @ 1.8V pulldown"
io8_ft_v33_fs_1v8  "IO8_FT_V33 fast speed @ 1.8V"
io8_ft_v33_fs_pu_1v8  "IO8_FT_V33 fast speed @ 1.8V pullup"
io8_ft_v33_fs_pd_1v8  "IO8_FT_V33 fast speed @ 1.8V pulldown"
io8_ft_v33_ms_1v8  "IO8_FT_V33 med speed @ 1.8V"
io8_ft_v33_ms_pu_1v8  "IO8_FT_V33 med speed @ 1.8V pullup"
io8_ft_v33_ms_pd_1v8  "IO8_FT_V33 med speed @ 1.8V pulldown"
io8_ft_v33_ls_1v8  "IO8_FT_V33 low speed @ 1.8V"
io8_ft_v33_ls_pu_1v8  "IO8_FT_V33 low speed @ 1.8V pullup"
io8_ft_v33_ls_pd_1v8  "IO8_FT_V33 low speed @ 1.8V pulldown"
io8_ft_v33_hs_3v3  "IO8_FT_V33 high speed @ 3.3V"
io8_ft_v33_hs_pu_3v3  "IO8_FT_V33 high speed @ 3.3V pullup"
io8_ft_v33_hs_pd_3v3  "IO8_FT_V33 high speed @ 3.3V pulldown"
io8_ft_v33_fs_3v3  "IO8_FT_V33 fast speed @ 3.3V"
io8_ft_v33_fs_pu_3v3  "IO8_FT_V33 fast speed @ 3.3V pullup"
io8_ft_v33_fs_pd_3v3  "IO8_FT_V33 fast speed @ 3.3V pulldown"
io8_ft_v33_ms_3v3  "IO8_FT_V33 med speed @ 3.3V"
io8_ft_v33_ms_pu_3v3  "IO8_FT_V33 med speed @ 3.3V pullup"
io8_ft_v33_ms_pd_3v3  "IO8_FT_V33 med speed @ 3.3V pulldown"
io8_ft_v33_ls_3v3  "IO8_FT_V33 low speed @ 3.3V"
io8_ft_v33_ls_pu_3v3  "IO8_FT_V33 low speed @ 3.3V pullup"
io8_ft_v33_ls_pd_3v3  "IO8_FT_V33 low speed @ 3.3V pulldown"
[Model Selector] io8_usb_ft
io8_100m_ft_hs_1v2  "IO8_FT 100MHz high speed @ 1.2V"
io8_100m_ft_hs_pu_1v2  "IO8_FT 100MHz high speed @ 1.2V pullup"
io8_100m_ft_hs_pd_1v2  "IO8_FT 100MHz high speed @ 1.2V pulldown"
io8_100m_ft_fs_1v2  "IO8_FT 100MHz fast speed @ 1.2V"
io8_100m_ft_fs_pu_1v2  "IO8_FT 100MHz fast speed @ 1.2V pullup"
io8_100m_ft_fs_pd_1v2  "IO8_FT 100MHz fast speed @ 1.2V pulldown"
io8_100m_ft_ms_1v2  "IO8_FT 100MHz med speed @ 1.2V"
io8_100m_ft_ms_pu_1v2  "IO8_FT 100MHz med speed @ 1.2V pullup"
io8_100m_ft_ms_pd_1v2  "IO8_FT 100MHz med speed @ 1.2V pulldown"
io8_100m_ft_ls_1v2  "IO8_FT 100MHz low speed @ 1.2V"
io8_100m_ft_ls_pu_1v2  "IO8_FT 100MHz low speed @ 1.2V pullup"
io8_100m_ft_ls_pd_1v2  "IO8_FT 100MHz low speed @ 1.2V pulldown"
io8_100m_ft_hs_1v8  "IO8_FT 100MHz high speed @ 1.8V"
io8_100m_ft_hs_pu_1v8  "IO8_FT 100MHz high speed @ 1.8V pullup"
io8_100m_ft_hs_pd_1v8  "IO8_FT 100MHz high speed @ 1.8V pulldown"
io8_100m_ft_fs_1v8  "IO8_FT 100MHz fast speed @ 1.8V"
io8_100m_ft_fs_pu_1v8  "IO8_FT 100MHz fast speed @ 1.8V pullup"
io8_100m_ft_fs_pd_1v8  "IO8_FT 100MHz fast speed @ 1.8V pulldown"
io8_100m_ft_ms_1v8  "IO8_FT 100MHz med speed @ 1.8V"
io8_100m_ft_ms_pu_1v8  "IO8_FT 100MHz med speed @ 1.8V pullup"
io8_100m_ft_ms_pd_1v8  "IO8_FT 100MHz med speed @ 1.8V pulldown"
io8_100m_ft_ls_1v8  "IO8_FT 100MHz low speed @ 1.8V"
io8_100m_ft_ls_pu_1v8  "IO8_FT 100MHz low speed @ 1.8V pullup"
io8_100m_ft_ls_pd_1v8  "IO8_FT 100MHz low speed @ 1.8V pulldown"
io8_100m_ft_hs_3v3  "IO8_FT 100MHz high speed @ 3.3V"
io8_100m_ft_hs_pu_3v3  "IO8_FT 100MHz high speed @ 3.3V pullup"
io8_100m_ft_hs_pd_3v3  "IO8_FT 100MHz high speed @ 3.3V pulldown"
io8_100m_ft_fs_3v3  "IO8_FT 100MHz fast speed @ 3.3V"
io8_100m_ft_fs_pu_3v3  "IO8_FT 100MHz fast speed @ 3.3V pullup"
io8_100m_ft_fs_pd_3v3  "IO8_FT 100MHz fast speed @ 3.3V pulldown"
io8_100m_ft_ms_3v3  "IO8_FT 100MHz med speed @ 3.3V"
io8_100m_ft_ms_pu_3v3  "IO8_FT 100MHz med speed @ 3.3V pullup"
io8_100m_ft_ms_pd_3v3  "IO8_FT 100MHz med speed @ 3.3V pulldown"
io8_100m_ft_ls_3v3  "IO8_FT 100MHz low speed @ 3.3V"
io8_100m_ft_ls_pu_3v3  "IO8_FT 100MHz low speed @ 3.3V pullup"
io8_100m_ft_ls_pd_3v3  "IO8_FT 100MHz low speed @ 3.3V pulldown"
io8_usb_fs_3v3  "IOUSB fast speed @ 3.3V"
io8_usb_fs_pu1_3v3  "IO8USB fast speed @ 3.3V pullup1"
io8_usb_fs_pd1_3v3  "IOUSB fast speed @ 3.3V pulldown1"
io8_usb_ls_3v3  "IOUSB low speed @ 3.3V"
io8_usb_ls_pu1_3v3  "IOUSB low speed @ 3.3V pullup1"
io8_usb_ls_pd1_3v3  "IOUSB low speed @ 3.3V pulldown1"
io8_usb_fs_pu2_3v3  "IOUSB fast speed @ 3.3V pullup2"
io8_usb_fs_pd2_3v3  "IOUSB fast speed @ 3.3V pulldown2"
io8_usb_ls_pu2_3v3  "IOUSB low speed @ 3.3V pullup2"
io8_usb_ls_pd2_3v3  "IOUSB low speed @ 3.3V pulldown2"
[Model Selector] io8_166m_hslv_ft
io8_166m_ft_hs_1v2  "IO8_FT 166MHz high speed @ 1.2V"
io8_166m_ft_hs_pu_1v2  "IO8_FT 166MHz high speed @ 1.2V pullup"
io8_166m_ft_hs_pd_1v2  "IO8_FT 166MHz high speed @ 1.2V pulldown"
io8_166m_ft_fs_1v2  "IO8_FT 166MHz fast speed @ 1.2V"
io8_166m_ft_fs_pu_1v2  "IO8_FT 166MHz fast speed @ 1.2V pullup"
io8_166m_ft_fs_pd_1v2  "IO8_FT 166MHz fast speed @ 1.2V pulldown"
io8_166m_ft_ms_1v2  "IO8_FT 166MHz med speed @ 1.2V"
io8_166m_ft_ms_pu_1v2  "IO8_FT 166MHz med speed @ 1.2V pullup"
io8_166m_ft_ms_pd_1v2  "IO8_FT 166MHz med speed @ 1.2V pulldown"
io8_166m_ft_ls_1v2  "IO8_FT 166MHz low speed @ 1.2V"
io8_166m_ft_ls_pu_1v2  "IO8_FT 166MHz low speed @ 1.2V pullup"
io8_166m_ft_ls_pd_1v2  "IO8_FT 166MHz low speed @ 1.2V pulldown"
io8_166m_ft_hs_1v8  "IO8_FT 166MHz high speed @ 1.8V"
io8_166m_ft_hs_pu_1v8  "IO8_FT 166MHz high speed @ 1.8V pullup"
io8_166m_ft_hs_pd_1v8  "IO8_FT 166MHz high speed @ 1.8V pulldown"
io8_166m_ft_fs_1v8  "IO8_FT 166MHz fast speed @ 1.8V"
io8_166m_ft_fs_pu_1v8  "IO8_FT 166MHz fast speed @ 1.8V pullup"
io8_166m_ft_fs_pd_1v8  "IO8_FT 166MHz fast speed @ 1.8V pulldown"
io8_166m_ft_ms_1v8  "IO8_FT 166MHz med speed @ 1.8V"
io8_166m_ft_ms_pu_1v8  "IO8_FT 166MHz med speed @ 1.8V pullup"
io8_166m_ft_ms_pd_1v8  "IO8_FT 166MHz med speed @ 1.8V pulldown"
io8_166m_ft_ls_1v8  "IO8_FT 166MHz low speed @ 1.8V"
io8_166m_ft_ls_pu_1v8  "IO8_FT 166MHz low speed @ 1.8V pullup"
io8_166m_ft_ls_pd_1v8  "IO8_FT 166MHz low speed @ 1.8V pulldown"
io8_166m_ft_hs_3v3  "IO8_FT 166MHz high speed @ 3.3V"
io8_166m_ft_hs_pu_3v3  "IO8_FT 166MHz high speed @ 3.3V pullup"
io8_166m_ft_hs_pd_3v3  "IO8_FT 166MHz high speed @ 3.3V pulldown"
io8_166m_ft_fs_3v3  "IO8_FT 166MHz fast speed @ 3.3V"
io8_166m_ft_fs_pu_3v3  "IO8_FT 166MHz fast speed @ 3.3V pullup"
io8_166m_ft_fs_pd_3v3  "IO8_FT 166MHz fast speed @ 3.3V pulldown"
io8_166m_ft_ms_3v3  "IO8_FT 166MHz med speed @ 3.3V"
io8_166m_ft_ms_pu_3v3  "IO8_FT 166MHz med speed @ 3.3V pullup"
io8_166m_ft_ms_pd_3v3  "IO8_FT 166MHz med speed @ 3.3V pulldown"
io8_166m_ft_ls_3v3  "IO8_FT 166MHz low speed @ 3.3V"
io8_166m_ft_ls_pu_3v3  "IO8_FT 166MHz low speed @ 3.3V pullup"
io8_166m_ft_ls_pd_3v3  "IO8_FT 166MHz low speed @ 3.3V pulldown"
io8_166m_hslv_ft_hs_1v2  "IO8_FT 166MHz HSLV high speed @ 1.2V"
io8_166m_hslv_ft_hs_pu_1v2  "IO8_FT 166MHz HSLV high speed @ 1.2V pullup"
io8_166m_hslv_ft_hs_pd_1v2  "IO8_FT 166MHz HSLV high speed @ 1.2V pulldown"
io8_166m_hslv_ft_fs_1v2  "IO8_FT 166MHz HSLV fast speed @ 1.2V"
io8_166m_hslv_ft_fs_pu_1v2  "IO8_FT 166MHz HSLV fast speed @ 1.2V pullup"
io8_166m_hslv_ft_fs_pd_1v2  "IO8_FT 166MHz HSLV fast speed @ 1.2V pulldown"
io8_166m_hslv_ft_ms_1v2  "IO8_FT 166MHz HSLV med speed @ 1.2V"
io8_166m_hslv_ft_ms_pu_1v2  "IO8_FT 166MHz HSLV med speed @ 1.2V pullup"
io8_166m_hslv_ft_ms_pd_1v2  "IO8_FT 166MHz HSLV med speed @ 1.2V pulldown"
io8_166m_hslv_ft_ls_1v2  "IO8_FT 166MHz HSLV low speed @ 1.2V"
io8_166m_hslv_ft_ls_pu_1v2  "IO8_FT 166MHz HSLV low speed @ 1.2V pullup"
io8_166m_hslv_ft_ls_pd_1v2  "IO8_FT 166MHz HSLV low speed @ 1.2V pulldown"
io8_166m_hslv_ft_hs_1v8  "IO8_FT 166MHz HSLV high speed @ 1.8V"
io8_166m_hslv_ft_hs_pu_1v8  "IO8_FT 166MHz HSLV high speed @ 1.8V pullup"
io8_166m_hslv_ft_hs_pd_1v8  "IO8_FT 166MHz HSLV high speed @ 1.8V pulldown"
io8_166m_hslv_ft_fs_1v8  "IO8_FT 166MHz HSLV fast speed @ 1.8V"
io8_166m_hslv_ft_fs_pu_1v8  "IO8_FT 166MHz HSLV fast speed @ 1.8V pullup"
io8_166m_hslv_ft_fs_pd_1v8  "IO8_FT 166MHz HSLV fast speed @ 1.8V pulldown"
io8_166m_hslv_ft_ms_1v8  "IO8_FT 166MHz HSLV med speed @ 1.8V"
io8_166m_hslv_ft_ms_pu_1v8  "IO8_FT 166MHz HSLV med speed @ 1.8V pullup"
io8_166m_hslv_ft_ms_pd_1v8  "IO8_FT 166MHz HSLV med speed @ 1.8V pulldown"
io8_166m_hslv_ft_ls_1v8  "IO8_FT 166MHz HSLV low speed @ 1.8V"
io8_166m_hslv_ft_ls_pu_1v8  "IO8_FT 166MHz HSLV low speed @ 1.8V pullup"
io8_166m_hslv_ft_ls_pd_1v8  "IO8_FT 166MHz HSLV low speed @ 1.8V pulldown"
io8_166m_hslv_ft_hs_2v5  "IO8_FT 166MHz HSLV high speed @ 2.5V"
io8_166m_hslv_ft_hs_pu_2v5  "IO8_FT 166MHz HSLV high speed @ 2.5V pullup"
io8_166m_hslv_ft_hs_pd_2v5  "IO8_FT 166MHz HSLV high speed @ 2.5V pulldown"
io8_166m_hslv_ft_fs_2v5  "IO8_FT 166MHz HSLV fast speed @ 2.5V"
io8_166m_hslv_ft_fs_pu_2v5  "IO8_FT 166MHz HSLV fast speed @ 2.5V pullup"
io8_166m_hslv_ft_fs_pd_2v5  "IO8_FT 166MHz HSLV fast speed @ 2.5V pulldown"
io8_166m_hslv_ft_ms_2v5  "IO8_FT 166MHz HSLV med speed @ 2.5V"
io8_166m_hslv_ft_ms_pu_2v5  "IO8_FT 166MHz HSLV med speed @ 2.5V pullup"
io8_166m_hslv_ft_ms_pd_2v5  "IO8_FT 166MHz HSLV med speed @ 2.5V pulldown"
io8_166m_hslv_ft_ls_2v5  "IO8_FT 166MHz HSLV low speed @ 2.5V"
io8_166m_hslv_ft_ls_pu_2v5  "IO8_FT 166MHz HSLV low speed @ 2.5V pullup"
io8_166m_hslv_ft_ls_pd_2v5  "IO8_FT 166MHz HSLV low speed @ 2.5V pulldown"
[Model Selector] io8_166m_hslv_i2c_ft
io8_166m_ft_hs_1v2  "IO8_FT 166MHz high speed @ 1.2V"
io8_166m_ft_hs_pu_1v2  "IO8_FT 166MHz high speed @ 1.2V pullup"
io8_166m_ft_hs_pd_1v2  "IO8_FT 166MHz high speed @ 1.2V pulldown"
io8_166m_ft_fs_1v2  "IO8_FT 166MHz fast speed @ 1.2V"
io8_166m_ft_fs_pu_1v2  "IO8_FT 166MHz fast speed @ 1.2V pullup"
io8_166m_ft_fs_pd_1v2  "IO8_FT 166MHz fast speed @ 1.2V pulldown"
io8_166m_ft_ms_1v2  "IO8_FT 166MHz med speed @ 1.2V"
io8_166m_ft_ms_pu_1v2  "IO8_FT 166MHz med speed @ 1.2V pullup"
io8_166m_ft_ms_pd_1v2  "IO8_FT 166MHz med speed @ 1.2V pulldown"
io8_166m_ft_ls_1v2  "IO8_FT 166MHz low speed @ 1.2V"
io8_166m_ft_ls_pu_1v2  "IO8_FT 166MHz low speed @ 1.2V pullup"
io8_166m_ft_ls_pd_1v2  "IO8_FT 166MHz low speed @ 1.2V pulldown"
io8_166m_ft_hs_1v8  "IO8_FT 166MHz high speed @ 1.8V"
io8_166m_ft_hs_pu_1v8  "IO8_FT 166MHz high speed @ 1.8V pullup"
io8_166m_ft_hs_pd_1v8  "IO8_FT 166MHz high speed @ 1.8V pulldown"
io8_166m_ft_fs_1v8  "IO8_FT 166MHz fast speed @ 1.8V"
io8_166m_ft_fs_pu_1v8  "IO8_FT 166MHz fast speed @ 1.8V pullup"
io8_166m_ft_fs_pd_1v8  "IO8_FT 166MHz fast speed @ 1.8V pulldown"
io8_166m_ft_ms_1v8  "IO8_FT 166MHz med speed @ 1.8V"
io8_166m_ft_ms_pu_1v8  "IO8_FT 166MHz med speed @ 1.8V pullup"
io8_166m_ft_ms_pd_1v8  "IO8_FT 166MHz med speed @ 1.8V pulldown"
io8_166m_ft_ls_1v8  "IO8_FT 166MHz low speed @ 1.8V"
io8_166m_ft_ls_pu_1v8  "IO8_FT 166MHz low speed @ 1.8V pullup"
io8_166m_ft_ls_pd_1v8  "IO8_FT 166MHz low speed @ 1.8V pulldown"
io8_166m_ft_hs_3v3  "IO8_FT 166MHz high speed @ 3.3V"
io8_166m_ft_hs_pu_3v3  "IO8_FT 166MHz high speed @ 3.3V pullup"
io8_166m_ft_hs_pd_3v3  "IO8_FT 166MHz high speed @ 3.3V pulldown"
io8_166m_ft_fs_3v3  "IO8_FT 166MHz fast speed @ 3.3V"
io8_166m_ft_fs_pu_3v3  "IO8_FT 166MHz fast speed @ 3.3V pullup"
io8_166m_ft_fs_pd_3v3  "IO8_FT 166MHz fast speed @ 3.3V pulldown"
io8_166m_ft_ms_3v3  "IO8_FT 166MHz med speed @ 3.3V"
io8_166m_ft_ms_pu_3v3  "IO8_FT 166MHz med speed @ 3.3V pullup"
io8_166m_ft_ms_pd_3v3  "IO8_FT 166MHz med speed @ 3.3V pulldown"
io8_166m_ft_ls_3v3  "IO8_FT 166MHz low speed @ 3.3V"
io8_166m_ft_ls_pu_3v3  "IO8_FT 166MHz low speed @ 3.3V pullup"
io8_166m_ft_ls_pd_3v3  "IO8_FT 166MHz low speed @ 3.3V pulldown"
io8_166m_hslv_ft_hs_1v2  "IO8_FT 166MHz HSLV high speed @ 1.2V"
io8_166m_hslv_ft_hs_pu_1v2  "IO8_FT 166MHz HSLV high speed @ 1.2V pullup"
io8_166m_hslv_ft_hs_pd_1v2  "IO8_FT 166MHz HSLV high speed @ 1.2V pulldown"
io8_166m_hslv_ft_fs_1v2  "IO8_FT 166MHz HSLV fast speed @ 1.2V"
io8_166m_hslv_ft_fs_pu_1v2  "IO8_FT 166MHz HSLV fast speed @ 1.2V pullup"
io8_166m_hslv_ft_fs_pd_1v2  "IO8_FT 166MHz HSLV fast speed @ 1.2V pulldown"
io8_166m_hslv_ft_ms_1v2  "IO8_FT 166MHz HSLV med speed @ 1.2V"
io8_166m_hslv_ft_ms_pu_1v2  "IO8_FT 166MHz HSLV med speed @ 1.2V pullup"
io8_166m_hslv_ft_ms_pd_1v2  "IO8_FT 166MHz HSLV med speed @ 1.2V pulldown"
io8_166m_hslv_ft_ls_1v2  "IO8_FT 166MHz HSLV low speed @ 1.2V"
io8_166m_hslv_ft_ls_pu_1v2  "IO8_FT 166MHz HSLV low speed @ 1.2V pullup"
io8_166m_hslv_ft_ls_pd_1v2  "IO8_FT 166MHz HSLV low speed @ 1.2V pulldown"
io8_166m_hslv_ft_hs_1v8  "IO8_FT 166MHz HSLV high speed @ 1.8V"
io8_166m_hslv_ft_hs_pu_1v8  "IO8_FT 166MHz HSLV high speed @ 1.8V pullup"
io8_166m_hslv_ft_hs_pd_1v8  "IO8_FT 166MHz HSLV high speed @ 1.8V pulldown"
io8_166m_hslv_ft_fs_1v8  "IO8_FT 166MHz HSLV fast speed @ 1.8V"
io8_166m_hslv_ft_fs_pu_1v8  "IO8_FT 166MHz HSLV fast speed @ 1.8V pullup"
io8_166m_hslv_ft_fs_pd_1v8  "IO8_FT 166MHz HSLV fast speed @ 1.8V pulldown"
io8_166m_hslv_ft_ms_1v8  "IO8_FT 166MHz HSLV med speed @ 1.8V"
io8_166m_hslv_ft_ms_pu_1v8  "IO8_FT 166MHz HSLV med speed @ 1.8V pullup"
io8_166m_hslv_ft_ms_pd_1v8  "IO8_FT 166MHz HSLV med speed @ 1.8V pulldown"
io8_166m_hslv_ft_ls_1v8  "IO8_FT 166MHz HSLV low speed @ 1.8V"
io8_166m_hslv_ft_ls_pu_1v8  "IO8_FT 166MHz HSLV low speed @ 1.8V pullup"
io8_166m_hslv_ft_ls_pd_1v8  "IO8_FT 166MHz HSLV low speed @ 1.8V pulldown"
io8_166m_hslv_ft_hs_2v5  "IO8_FT 166MHz HSLV high speed @ 2.5V"
io8_166m_hslv_ft_hs_pu_2v5  "IO8_FT 166MHz HSLV high speed @ 2.5V pullup"
io8_166m_hslv_ft_hs_pd_2v5  "IO8_FT 166MHz HSLV high speed @ 2.5V pulldown"
io8_166m_hslv_ft_fs_2v5  "IO8_FT 166MHz HSLV fast speed @ 2.5V"
io8_166m_hslv_ft_fs_pu_2v5  "IO8_FT 166MHz HSLV fast speed @ 2.5V pullup"
io8_166m_hslv_ft_fs_pd_2v5  "IO8_FT 166MHz HSLV fast speed @ 2.5V pulldown"
io8_166m_hslv_ft_ms_2v5  "IO8_FT 166MHz HSLV med speed @ 2.5V"
io8_166m_hslv_ft_ms_pu_2v5  "IO8_FT 166MHz HSLV med speed @ 2.5V pullup"
io8_166m_hslv_ft_ms_pd_2v5  "IO8_FT 166MHz HSLV med speed @ 2.5V pulldown"
io8_166m_hslv_ft_ls_2v5  "IO8_FT 166MHz HSLV low speed @ 2.5V"
io8_166m_hslv_ft_ls_pu_2v5  "IO8_FT 166MHz HSLV low speed @ 2.5V pullup"
io8_166m_hslv_ft_ls_pd_2v5  "IO8_FT 166MHz HSLV low speed @ 2.5V pulldown"
io8_166m_i2c_ft_1v2  "IO8_FT 166MHz I2C @ 1.2V"
io8_166m_i2c_ft_pu_1v2  "IO8_FT 166MHz I2C @ 1.2V pullup"
io8_166m_i2c_ft_pd_1v2  "IO8_FT 166MHz I2C @ 1.2V pulldown"
io8_166m_i2c_ft_1v8  "IO8_FT 166MHz I2C @ 1.8V"
io8_166m_i2c_ft_pu_1v8  "IO8_FT 166MHz I2C @ 1.8V pullup"
io8_166m_i2c_ft_pd_1v8  "IO8_FT 166MHz I2C @ 1,8V pulldown"
io8_166m_i2c_ft_3v3  "IO8_FT 166MHz I2C @ 3.3V"
io8_166m_i2c_ft_pu_3v3  "IO8_FT 166MHz I2C HSLV @ 3.3V pullup"
io8_166m_i2c_ft_pd_3v3  "IO8_FT 166MHz I2C @ 3.3V pulldown"
[Model Selector] io8_100m_ft_v33
io8_ft_v33_hs_1v2  "IO8_FT_V33 high speed @ 1.2V"
io8_ft_v33_hs_pu_1v2  "IO8_FT_V33 high speed @ 1.2V pullup"
io8_ft_v33_hs_pd_1v2  "IO8_FT_V33 high speed @ 1.2V pulldown"
io8_ft_v33_fs_1v2  "IO8_FT_V33 fast speed @ 1.2V"
io8_ft_v33_fs_pu_1v2  "IO8_FT_V33 fast speed @ 1.2V pullup"
io8_ft_v33_fs_pd_1v2  "IO8_FT_V33 fast speed @ 1.2V pulldown"
io8_ft_v33_ms_1v2  "IO8_FT_V33 med speed @ 1.2V"
io8_ft_v33_ms_pu_1v2  "IO8_FT_V33 med speed @ 1.2V pullup"
io8_ft_v33_ms_pd_1v2  "IO8_FT_V33 med speed @ 1.2V pulldown"
io8_ft_v33_ls_1v2  "IO8_FT_V33 low speed @ 1.2V"
io8_ft_v33_ls_pu_1v2  "IO8_FT_V33 low speed @ 1.2V pullup"
io8_ft_v33_ls_pd_1v2  "IO8_FT_V33 low speed @ 1.2V pulldown"
io8_ft_v33_hs_1v8  "IO8_FT_V33 high speed @ 1.8V"
io8_ft_v33_hs_pu_1v8  "IO8_FT_V33 high speed @ 1.8V pullup"
io8_ft_v33_hs_pd_1v8  "IO8_FT_V33 high speed @ 1.8V pulldown"
io8_ft_v33_fs_1v8  "IO8_FT_V33 fast speed @ 1.8V"
io8_ft_v33_fs_pu_1v8  "IO8_FT_V33 fast speed @ 1.8V pullup"
io8_ft_v33_fs_pd_1v8  "IO8_FT_V33 fast speed @ 1.8V pulldown"
io8_ft_v33_ms_1v8  "IO8_FT_V33 med speed @ 1.8V"
io8_ft_v33_ms_pu_1v8  "IO8_FT_V33 med speed @ 1.8V pullup"
io8_ft_v33_ms_pd_1v8  "IO8_FT_V33 med speed @ 1.8V pulldown"
io8_ft_v33_ls_1v8  "IO8_FT_V33 low speed @ 1.8V"
io8_ft_v33_ls_pu_1v8  "IO8_FT_V33 low speed @ 1.8V pullup"
io8_ft_v33_ls_pd_1v8  "IO8_FT_V33 low speed @ 1.8V pulldown"
io8_ft_v33_hs_3v3  "IO8_FT_V33 high speed @ 3.3V"
io8_ft_v33_hs_pu_3v3  "IO8_FT_V33 high speed @ 3.3V pullup"
io8_ft_v33_hs_pd_3v3  "IO8_FT_V33 high speed @ 3.3V pulldown"
io8_ft_v33_fs_3v3  "IO8_FT_V33 fast speed @ 3.3V"
io8_ft_v33_fs_pu_3v3  "IO8_FT_V33 fast speed @ 3.3V pullup"
io8_ft_v33_fs_pd_3v3  "IO8_FT_V33 fast speed @ 3.3V pulldown"
io8_ft_v33_ms_3v3  "IO8_FT_V33 med speed @ 3.3V"
io8_ft_v33_ms_pu_3v3  "IO8_FT_V33 med speed @ 3.3V pullup"
io8_ft_v33_ms_pd_3v3  "IO8_FT_V33 med speed @ 3.3V pulldown"
io8_ft_v33_ls_3v3  "IO8_FT_V33 low speed @ 3.3V"
io8_ft_v33_ls_pu_3v3  "IO8_FT_V33 low speed @ 3.3V pullup"
io8_ft_v33_ls_pd_3v3  "IO8_FT_V33 low speed @ 3.3V pulldown"
[Define Package Model]  455-lqfp-14x14-100-ldo-230504
[Manufacturer]  Unknown
[OEM]  Unknown
[Description]  None
[Number Of Pins]  96
[Pin Numbers]
| Pin Num   Terminal Name
14 | NRST
23 | PA0
69 | PA10
70 | PA11
71 | PA12
72 | PA13
76 | PA14
77 | PA15
24 | PA1
25 | PA2
26 | PA3
29 | PA4
30 | PA5
31 | PA6
32 | PA7
67 | PA8
68 | PA9
35 | PB0
47 | PB10
51 | PB12
52 | PB13
53 | PB14
54 | PB15
36 | PB1
37 | PB2
89 | PB3
90 | PB4
91 | PB5
92 | PB6
93 | PB7
95 | PB8
96 | PB9
15 | PC0
78 | PC10
79 | PC11
80 | PC12
7 | PC13
8 | PC14-OSC32_IN
9 | PC15-OSC32_OUT
16 | PC1
17 | PC2
18 | PC3
33 | PC4
34 | PC5
63 | PC6
64 | PC7
65 | PC8
66 | PC9
81 | PD0
57 | PD10
58 | PD11
59 | PD12
60 | PD13
61 | PD14
62 | PD15
82 | PD1
83 | PD2
84 | PD3
85 | PD4
86 | PD5
87 | PD6
88 | PD7
55 | PD8
56 | PD9
97 | PE0
41 | PE10
42 | PE11
43 | PE12
44 | PE13
45 | PE14
46 | PE15
98 | PE1
1 | PE2
2 | PE3
3 | PE4
4 | PE5
5 | PE6
38 | PE7
39 | PE8
40 | PE9
12 | PH0-OSC_IN
13 | PH1-OSC_OUT
94 | PH3-BOOT0
48 | VCAP
6 | VBAT
50 | VDD
75 | VDD
100 | VDD
28 | VDD
11 | VDD
73 | VDDUSB
22 | VDDA
20 | VREFM
21 | VREFP
10 | VSS
19 | VSSA
|[Merged Pins]  10
|27  |  VSS
|49  |  VSS
|74  |  VSS
|99  |  VSS
[Model Data]
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[End Model Data]
[End Package Model]
| Models and submodels in the file (208): io8_100m_ft_hs_1v2 (I/O), io8_100m_ft_hs_pu_1v2 (I/O), io8_100m_ft_hs_pd_1v2 (I/O), io8_100m_ft_fs_1v2 (I/O), io8_100m_ft_fs_pu_1v2 (I/O), io8_100m_ft_fs_pd_1v2 (I/O), io8_100m_ft_ms_1v2 (I/O), io8_100m_ft_ms_pu_1v2 (I/O), io8_100m_ft_ms_pd_1v2 (I/O), io8_100m_ft_ls_1v2 (I/O), io8_100m_ft_ls_pu_1v2 (I/O), io8_100m_ft_ls_pd_1v2 (I/O), io8_100m_ft_hs_1v8 (I/O), io8_100m_ft_hs_pu_1v8 (I/O), io8_100m_ft_hs_pd_1v8 (I/O), io8_100m_ft_fs_1v8 (I/O), io8_100m_ft_fs_pu_1v8 (I/O), io8_100m_ft_fs_pd_1v8 (I/O), io8_100m_ft_ms_1v8 (I/O), io8_100m_ft_ms_pu_1v8 (I/O), io8_100m_ft_ms_pd_1v8 (I/O), io8_100m_ft_ls_1v8 (I/O), io8_100m_ft_ls_pu_1v8 (I/O), io8_100m_ft_ls_pd_1v8 (I/O), io8_100m_ft_hs_3v3 (I/O), io8_100m_ft_hs_pu_3v3 (I/O), io8_100m_ft_hs_pd_3v3 (I/O), io8_100m_ft_fs_3v3 (I/O), io8_100m_ft_fs_pu_3v3 (I/O), io8_100m_ft_fs_pd_3v3 (I/O), io8_100m_ft_ms_3v3 (I/O), io8_100m_ft_ms_pu_3v3 (I/O), io8_100m_ft_ms_pd_3v3 (I/O), io8_100m_ft_ls_3v3 (I/O), io8_100m_ft_ls_pu_3v3 (I/O), io8_100m_ft_ls_pd_3v3 (I/O), io8_100m_hslv_ft_hs_1v2 (I/O), io8_100m_hslv_ft_hs_pu_1v2 (I/O), io8_100m_hslv_ft_hs_pd_1v2 (I/O), io8_100m_hslv_ft_fs_1v2 (I/O), io8_100m_hslv_ft_fs_pu_1v2 (I/O), io8_100m_hslv_ft_fs_pd_1v2 (I/O), io8_100m_hslv_ft_ms_1v2 (I/O), io8_100m_hslv_ft_ms_pu_1v2 (I/O), io8_100m_hslv_ft_ms_pd_1v2 (I/O), io8_100m_hslv_ft_ls_1v2 (I/O), io8_100m_hslv_ft_ls_pu_1v2 (I/O), io8_100m_hslv_ft_ls_pd_1v2 (I/O), io8_100m_hslv_ft_hs_1v8 (I/O), io8_100m_hslv_ft_hs_pu_1v8 (I/O), io8_100m_hslv_ft_hs_pd_1v8 (I/O), io8_100m_hslv_ft_fs_1v8 (I/O), io8_100m_hslv_ft_fs_pu_1v8 (I/O), io8_100m_hslv_ft_fs_pd_1v8 (I/O), io8_100m_hslv_ft_ms_1v8 (I/O), io8_100m_hslv_ft_ms_pu_1v8 (I/O), io8_100m_hslv_ft_ms_pd_1v8 (I/O), io8_100m_hslv_ft_ls_1v8 (I/O), io8_100m_hslv_ft_ls_pu_1v8 (I/O), io8_100m_hslv_ft_ls_pd_1v8 (I/O), io8_100m_hslv_ft_hs_2v5 (I/O), io8_100m_hslv_ft_hs_pu_2v5 (I/O), io8_100m_hslv_ft_hs_pd_2v5 (I/O), io8_100m_hslv_ft_fs_2v5 (I/O), io8_100m_hslv_ft_fs_pu_2v5 (I/O), io8_100m_hslv_ft_fs_pd_2v5 (I/O), io8_100m_hslv_ft_ms_2v5 (I/O), io8_100m_hslv_ft_ms_pu_2v5 (I/O), io8_100m_hslv_ft_ms_pd_2v5 (I/O), io8_100m_hslv_ft_ls_2v5 (I/O), io8_100m_hslv_ft_ls_pu_2v5 (I/O), io8_100m_hslv_ft_ls_pd_2v5 (I/O), io8_166m_ft_hs_1v2 (I/O), io8_166m_ft_hs_pu_1v2 (I/O), io8_166m_ft_hs_pd_1v2 (I/O), io8_166m_ft_fs_1v2 (I/O), io8_166m_ft_fs_pu_1v2 (I/O), io8_166m_ft_fs_pd_1v2 (I/O), io8_166m_ft_ms_1v2 (I/O), io8_166m_ft_ms_pu_1v2 (I/O)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
